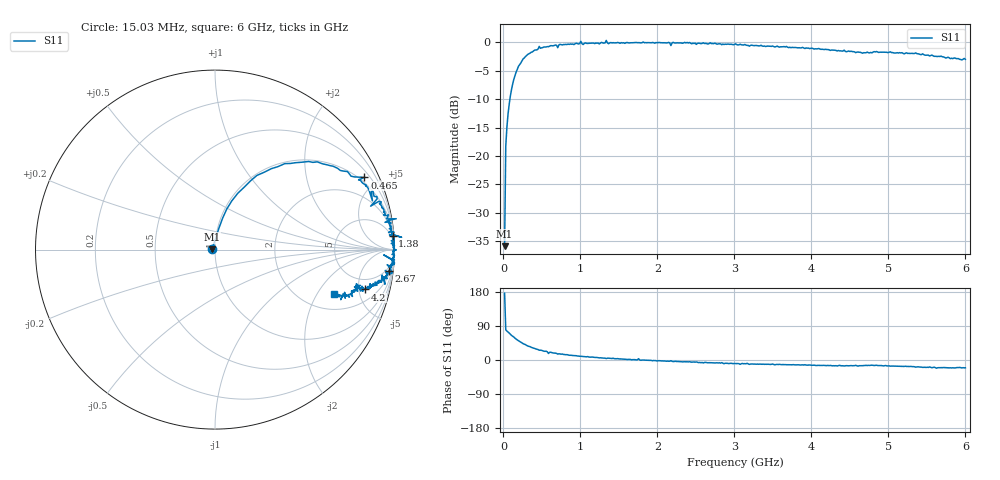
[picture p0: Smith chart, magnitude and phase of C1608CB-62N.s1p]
!	Network	Analyzer	HP8753E.07.74:	Oct	30	2002	Serial	No.	JP38451487
!	Hewlett-Packard
!	28	Aug	2009	8:21:51
!	Frequency	S11
#	HZ	S	RI	R	50
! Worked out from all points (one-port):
!   400 points, 15.03 MHz to 6 GHz, reference 50 ohm
!   lowest |S11| = -35.9 dB at 15.03 MHz (marker M1), VSWR 1.03, Z = 48.4 + j0.0998 ohm
!   |S11| at or under -10 dB: start of sweep to 83.86 MHz
!   S11 on the Smith chart (normalised r, x): 15.03 MHz: 0.97, +0.00; 465 MHz: 0.77, +4.24; 1.38 GHz: 3, +26; 2.67 GHz: 3, -16; 4.2 GHz: 3.29, -5.88; 6 GHz: 2.83, -2.86
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1.502992e7  -0.016 0.00103
3.002985e7  0.0221 0.12
6.00297e7  0.0656 0.226
9.002955e7  0.127 0.314
1.95029e8  0.389 0.479
4.650277e8  0.832 0.402
5.550272e8  0.839 0.361
5.850271e8  0.877 0.272
6.150269e8  0.88 0.326
7.650262e8  0.916 0.258
1.005025e9  1.01 0.172
1.035025e9  0.947 0.152
1.335023e9  1.04 0.0684
1.380023e9  0.989 0.0754
1.515022e9  0.982 0.0495
1.725021e9  1 0.0061
1.755021e9  0.995 0.0599
1.785021e9  0.992 -0.0131
2.145019e9  1 -0.0579
2.175019e9  0.94 -0.0295
2.265019e9  0.992 -0.0663
2.670017e9  0.97 -0.121
3.015015e9  0.96 -0.161
3.765011e9  0.883 -0.191
4.200009e9  0.838 -0.222
4.515007e9  0.81 -0.213
5.265004e9  0.767 -0.236
6e9  0.665 -0.25
